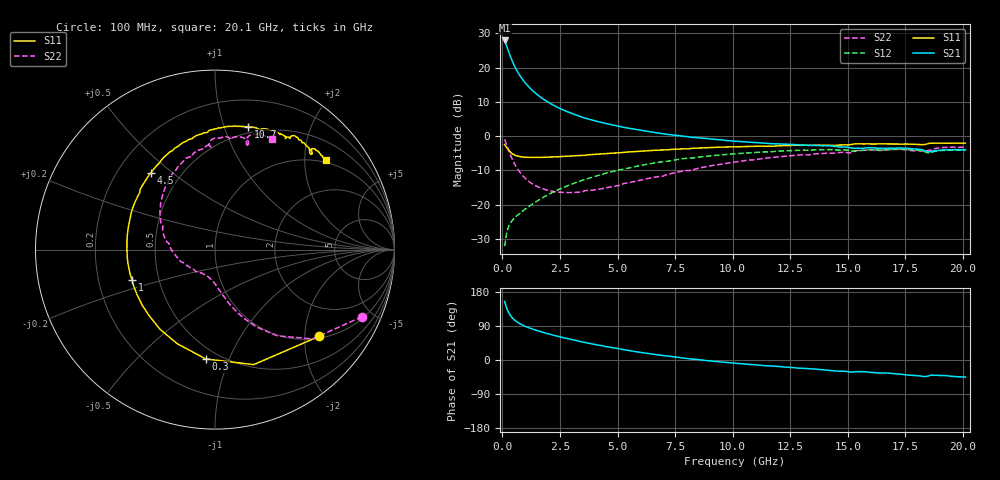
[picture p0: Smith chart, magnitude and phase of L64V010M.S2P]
!  Infineon Technologies AG
! BFR380L3 , PF131585-7, No.6, Th 09.10.01, soldered on pcb-board, measured with PP GSG850
!  Vce=4.0 V,  Ic=10.0 mA
! Common Emitter S-Parameters:  15. November 2001
#  GHz  S  MA  R  50
! f  S11  S21  S12  S22
! GHz  Mag  Ang  Mag  Ang  Mag  Ang  Mag  Ang
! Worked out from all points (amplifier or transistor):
!   201 points, 100 MHz to 20.1 GHz, reference 50 ohm
!   highest |S21| = 27.9 dB at 100 MHz (marker M1)
!   |S21| within 3 dB of that: start of sweep to 261.1 MHz
!   unconditionally stable (mu >= 1): 1.87 GHz to 4.493 GHz
!   at 3.4 GHz: K = 1.03, MAG = 8.3 dB, |S12| = -13.0 dB
!   at 10.1 GHz: K = 0.94, MSG = 1.8 dB, |S12| = -5.1 dB
!   at 20.1 GHz: K = 0.99, MSG = 0.0 dB, |S12| = -4.0 dB
!   S11 on the Smith chart (normalised r, x): 100 MHz: 1.05, -2.36; 300 MHz: 0.42, -0.82; 1 GHz: 0.35, -0.16; 4.5 GHz: 0.34, +0.42; 10.7 GHz: 0.44, +1.21; 20.1 GHz: 0.95, +2.53
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0.1  0.7556 -39.7  24.94 154.2  0.0249 71.0  0.9002 -24.6
0.2  0.6761 -71.4  20.21 135.1  0.04067 59.1  0.7367 -42.5
0.3  0.6112 -94.9  16.2 122.5  0.05073 52.9  0.594 -54.0
0.4  0.5649 -111.9  13.25 113.6  0.05707 49.7  0.4895 -61.8
0.5  0.5393 -124.7  11.09 107.1  0.06267 49.1  0.415 -67.2
0.6  0.5199 -134.8  9.5 102.1  0.06769 49.3  0.3604 -71.3
0.7  0.5101 -142.7  8.297 98.0  0.07223 49.8  0.319 -74.6
0.8  0.5021 -149.3  7.348 94.5  0.07691 50.7  0.2873 -77.3
1  0.4926 -159.9  5.981 88.8  0.08679 52.4  0.2428 -81.8
1.2  0.4909 -168.0  5.042 83.9  0.09697 54.0  0.2135 -85.7
1.4  0.4907 -174.4  4.36 79.8  0.1076 55.1  0.1931 -89.4
1.6  0.4907 179.5  3.843 75.9  0.1184 56.1  0.1791 -93.0
1.9  0.4942 172.1  3.276 70.6  0.1353 56.8  0.165 -98.2
2.6  0.5062 158.4  2.451 59.7  0.1755 56.6  0.1517 -111.7
3.5  0.5249 143.4  1.88 47.3  0.2294 53.9  0.1556 -128.0
4.5  0.5579 129.7  1.529 35.4  0.2888 49.4  0.1765 -148.6
6.8  0.6262 104.5  1.109 13.0  0.4178 35.5  0.258 173.0
10.1  0.7007 78.9  0.8461 -8.3  0.5547 13.9  0.4205 134.1
10.7  0.7102 74.8  0.8178 -11.5  0.5736 9.8  0.4482 127.4
13.5  0.7364 60.5  0.7386 -23.7  0.6297 -7.7  0.5462 102.9
16.8  0.7699 48.2  0.6702 -34.7  0.6366 -24.3  0.6375 79.9
20.1  0.7927 38.8  0.6357 -45.2  0.6285 -38.4  0.6924 62.7
